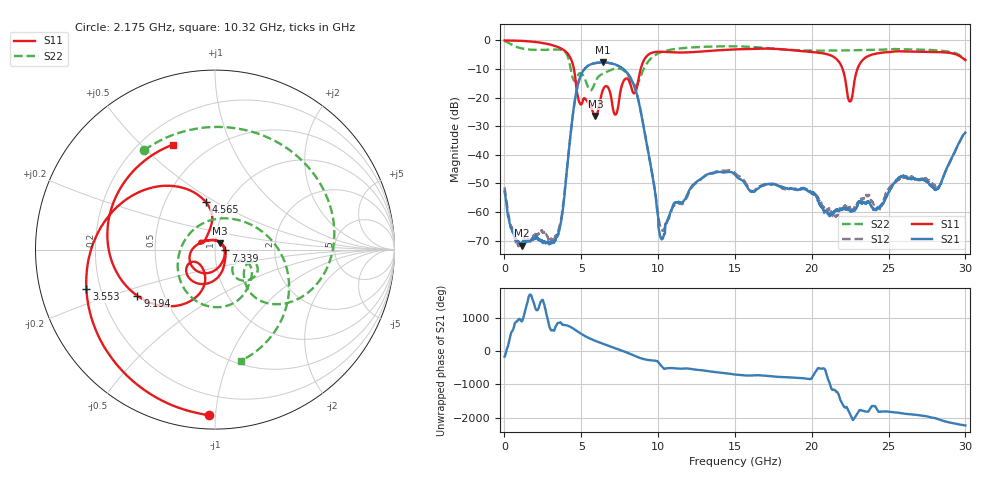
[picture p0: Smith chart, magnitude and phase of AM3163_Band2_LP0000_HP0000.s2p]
!Agilent Technologies,E8364B,MY43040894,A.07.50.67
!Agilent E8364B: A.07.50.67
!Date: Thursday, August 20, 2020 11:09:59
!Correction: S11(Full 2 Port(1,2))
!S21(Full 2 Port(1,2))
!S12(Full 2 Port(1,2))
!S22(Full 2 Port(1,2))
!S2P File: Measurements: S11, S21, S12, S22:
# Hz S  dB  R 50
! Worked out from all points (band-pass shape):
!   3201 points, 10 MHz to 30 GHz, reference 50 ohm
!   highest |S21| = -7.71 dB at 6.402 GHz (marker M1); lowest = -71.8 dB at 1.135 GHz (marker M2)
!   |S21| within 3 dB of the highest: 5.118 GHz to 7.877 GHz (2.759 GHz wide, 42.5 % of centre)
!   lowest |S11| = -26.5 dB at 5.914 GHz (marker M3), VSWR 1.10, Z = 52.8 + j3.96 ohm
!   |S11| at or under -10 dB: 4.521 GHz to 8.868 GHz (4.347 GHz wide, 64.9 % of centre); 22.01 GHz to 22.98 GHz (969 MHz wide, 4.31 % of centre)
!   |S22| runs from -17.5 to -0.3 dB; largest |S21 - S12| = 0.0041
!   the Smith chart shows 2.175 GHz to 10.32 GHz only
!   S11 on the Smith chart (normalised r, x): 2.175 GHz: 0.08, -0.96; 3.553 GHz: 0.15, -0.15; 4.565 GHz: 0.79, +0.45; 7.339 GHz: 1.12, -0.01; 9.194 GHz: 0.35, -0.24; 10.32 GHz: 0.32, +0.62
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1e7  -0.05 -3.0  -52.89 -161.6  -51.41 -53.7  -0.29 -12.5
5.067094e8  -0.07 -20.9  -66.89 -107.4  -66.21 115.6  -1.64 -82.9
1.134625e9  -0.18 -47.1  -71.79 -178.8  -70.68 -179.3  -2.83 -153.6
2.174903e9  -0.69 -92.2  -69.72 171.7  -67.74 139.2  -3.35 125.6
3.552569e9  -2.50 -162.9  -66.70 137.4  -65.75 -63.5  -3.22 27.6
4.564731e9  -11.33 101.2  -21.62 -60.9  -21.64 -61.1  -14.24 -30.8
5.014581e9  -22.35 148.8  -11.72 159.7  -11.73 159.4  -11.64 -37.7
5.914281e9  -26.49 52.1  -7.96 -46.4  -7.96 -46.6  -14.54 -20.9
6.401619e9  -17.44 -104.9  -7.71 -133.1  -7.71 -133.2  -11.68 -40.4
7.338806e9  -24.81 -5.0  -8.72 71.4  -8.77 71.3  -9.85 -84.1
9.194438e9  -5.96 -149.2  -34.31 109.8  -34.21 109.7  -8.73 -3.0
1.000979e10  -3.99 136.3  -62.19 33.8  -61.54 142.9  -4.58 -61.4
1.031906e10  -4.01 112.1  -69.06 -134.8  -66.34 125.6  -3.92 -77.0
1.208098e10  -4.17 -7.9  -52.01 -171.0  -52.28 -166.0  -2.52 -142.5
1.5005e10  -3.16 -144.3  -47.05 16.8  -46.39 17.5  -2.09 124.9
1.768536e10  -2.99 93.8  -50.53 -50.1  -50.30 -49.7  -2.99 27.1
2.000958e10  -4.09 -30.9  -53.48 -82.9  -53.58 -125.8  -3.60 -52.4
2.172463e10  -7.18 -124.0  -59.61 154.9  -60.42 -133.3  -3.58 -101.4
2.248376e10  -21.41 -104.6  -59.40 -91.2  -58.36 97.0  -3.51 -121.1
2.500479e10  -4.11 -151.5  -52.94 -27.0  -51.88 -20.7  -3.20 177.7
2.825683e10  -4.11 107.2  -51.51 109.7  -51.25 106.9  -3.54 90.9
3e10  -6.92 42.4  -32.32 -79.9  -32.05 -79.4  -6.79 37.4
